(* Logix 5000 AddOnInstructionDefinition export AMCI_SV160E2_Immediate_Stop; software revision 20.03 *)

ADD_ON_INSTRUCTION AMCI_SV160E2_Immediate_Stop   (* revision 1.0, vendor AMCI *)
// Revision note:
// 8/2019 Version 0 Initial release of SV160E2 Add On Instructions.
// 3/17/20 Version 1 replaced the generic EDS file with a more complete V1.6 EDS file.
VAR_IN_OUT
   AMCI_SV160E2_OUTPUT_DATA : _000A:SV160E2_9125ACD4:O:0; {required}
END_VAR
VAR
   command_data_block : INT[10];
        [0]   // Command Bits MSW
        [1]   // Command Bits LSW
        [2]   // Upper Target Position
        [3]   // Lower Target Position
        [4]   // Upper Programmed Speed
        [5]   // Lower Programmed Speed
END_VAR

ROUTINE Logic   (* ladder *)
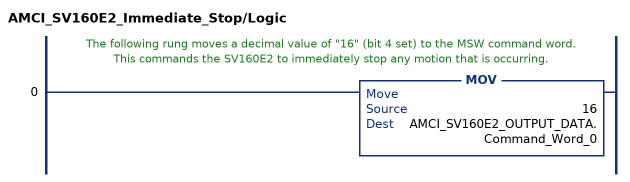
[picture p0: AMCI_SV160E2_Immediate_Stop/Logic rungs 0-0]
   // The following rung moves a decimal value of "16" (bit 4 set) to the MSW command word.  This commands the SV160E2 to immediately stop any motion that is occurring.
   0: MOV(16,AMCI_SV160E2_OUTPUT_DATA.Command_Word_0);
END_ROUTINE
END_ADD_ON_INSTRUCTION
